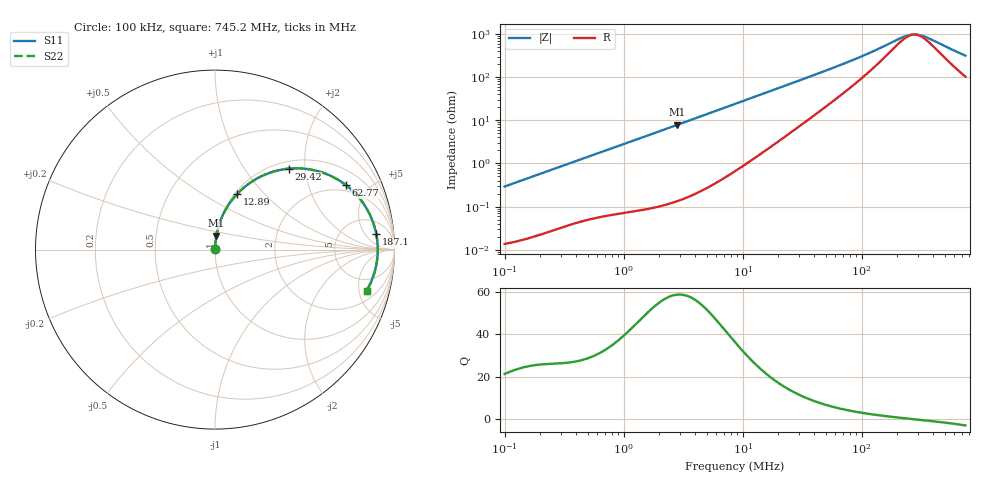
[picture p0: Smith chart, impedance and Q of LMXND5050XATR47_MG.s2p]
! LMXND5050XATR47_MG  S-PARAMETER MODEL  ( General Type )
! Model Generated by TAIYO YUDEN Corporation (http://www.ty-top.com)
! Version 1.0
! TAIYO YUDEN Control No. 191023NI43SB-FBB
! Copyright(c) 2019 TAIYO YUDEN CO.,LTD. All Rights Reserved.
! Product Description (link to TY-COMPAS)
! https://ds.yuden.co.jp/TYCOMPAS/or/detail?pn=LMXND5050XATR47NMG&u=M
! Products Name : Inductors
! Characteristics :
!  Inductance : 0.47 uH , SRF(min) : 185 MHz , DC Resistance(max) : 0.013 Ohm
!  Rated Current : Saturation :9000 mA , Temp Rise : 5000 mA
!  Case Size : 4.9 x 4.9 / 0.193 x 0.193 [mm/inch] , Thickness : 3.1 / 0.122 [mm/inch]
!  (Conditions: Temperature = 25 degC , DC Bias Current/Voltage = 0A / 0V)
! External Node Assignments :
!  1  o---GGG---o  2
! GND o---------o GND
! Frequency Range : 0.1MHz  -  745.243127MHz  [ 402 STEP ]
# MHz S RI R 50
! Freq[MHz].  S11 Real  S11 Imag  S21 Real  S21 Imag  S12 Real  S12 Imag  S22 Real  S22 Imag
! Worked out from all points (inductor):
!   401 points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, 100 kHz to 745.2 MHz, reference 50 ohm
!   read as one part in series: L = 462 nH near 104.6 kHz
!   highest Q = 58.7 at 2.832 MHz (marker M1), where L = 441 nH
!   self-resonance near 278.1 MHz
!   S11 on the Smith chart (normalised r, x): 100 kHz: 1.00, +0.01; 12.89 MHz: 1.03, +0.71; 29.42 MHz: 1.14, +1.63; 62.77 MHz: 1.67, +3.53; 187.1 MHz: 10, +10; 745.2 MHz: 3.04, -5.97
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0.1  0.000145 0.00291  0.9999 -0.00291  0.9999 -0.00291  0.000145 0.00291
0.445256  0.000612 0.0126  0.9994 -0.0126  0.9994 -0.0126  0.000612 0.0126
1.98253  0.004 0.0547  0.996 -0.0547  0.996 -0.0547  0.004 0.0547
2.832121  0.00742 0.0778  0.9926 -0.0778  0.9926 -0.0778  0.00742 0.0778
5.056047  0.0218 0.1365  0.9782 -0.1365  0.9782 -0.1365  0.0218 0.1365
8.632747  0.0595 0.2232  0.9405 -0.2232  0.9405 -0.2232  0.0595 0.2232
12.89444  0.1225 0.309  0.8775 -0.309  0.8775 -0.309  0.1225 0.309
19.25998  0.2347 0.3966  0.7653 -0.3966  0.7653 -0.3966  0.2347 0.3966
29.41643  0.4097 0.4509  0.5903 -0.4509  0.5903 -0.4509  0.4097 0.4509
38.43783  0.5335 0.446  0.4665 -0.446  0.4665 -0.446  0.5335 0.446
48.03595  0.6305 0.4172  0.3695 -0.4172  0.3695 -0.4172  0.6305 0.4172
62.76757  0.728 0.3607  0.272 -0.3607  0.272 -0.3607  0.728 0.3607
100.2377  0.8389 0.2386  0.1611 -0.2386  0.1611 -0.2386  0.8389 0.2386
171.1468  0.8942 0.1064  0.1058 -0.1064  0.1058 -0.1064  0.8942 0.1064
187.1078  0.8986 0.0861  0.1014 -0.0861  0.1014 -0.0861  0.8986 0.0861
223.634  0.9044 0.0468  0.0956 -0.0468  0.0956 -0.0468  0.9044 0.0468
250.0008  0.9063 0.0228  0.0937 -0.0228  0.0937 -0.0228  0.9063 0.0228
279.4764  0.9069 -0.0011  0.0931 0.0011  0.0931 0.0011  0.9069 -0.0011
305.5401  0.9064 -0.0202  0.0936 0.0202  0.0936 0.0202  0.9064 -0.0202
357.1358  0.9037 -0.0539  0.0963 0.0539  0.0963 0.0539  0.9037 -0.0539
583.1896  0.8749 -0.1672  0.1251 0.1672  0.1251 0.1672  0.8749 -0.1672
745.2431  0.8444 -0.2297  0.1556 0.2297  0.1556 0.2297  0.8444 -0.2297
